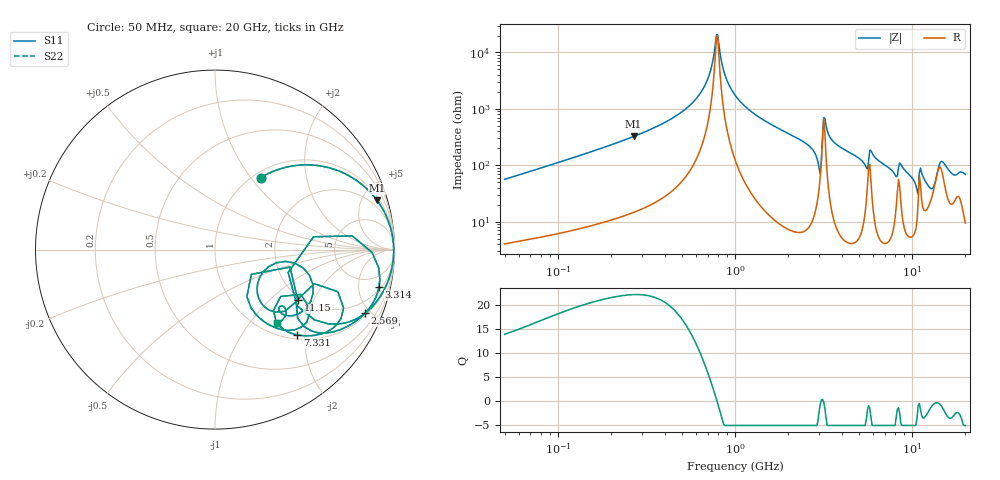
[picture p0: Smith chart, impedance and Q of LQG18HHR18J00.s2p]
!Murata Part Number: LQG18HHR18J00
!These Parameters are Measured in Series Mode Connection
!  o--[Z]--o
!Port1  Port2
!  o-------o
!Freq. Start=50[MHz] Stop=20[GHz], 401[Steps]
# Hz S RI R 50
!Freq.(Hz) S11(Real) S11(Imag) S21(Real) S21(Imag) S12(Real) S12(Imag) S22(Real) S22(Imag)
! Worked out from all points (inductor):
!   401 points, 50 MHz to 20 GHz, reference 50 ohm
!   read as one part in series: L = 176 nH near 51.52 MHz
!   highest Q = 22.2 at 267.6 MHz (marker M1), where L = 192 nH
!   self-resonance near 786.9 MHz
!   S11 on the Smith chart (normalised r, x): 50 MHz: 1.08, +1.12; 2.569 GHz: 1.15, -4.63; 3.314 GHz: 2.41, -8.24; 7.331 GHz: 1.09, -1.83; 11.15 GHz: 1.91, -1.53; 20 GHz: 1.19, -1.37
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5e7  0.2552 0.4016  0.7448 -0.4016  0.7448 -0.4016  0.2552 0.4016
1.364002e8  0.6917 0.4374  0.3083 -0.4374  0.3083 -0.4374  0.6917 0.4374
2.676374e8  0.9027 0.2747  0.0973 -0.2747  0.0973 -0.2747  0.9027 0.2747
3.721004e8  0.9546 0.1859  0.0454 -0.1859  0.0454 -0.1859  0.9546 0.1859
6.380365e8  0.9921 0.0514  0.00789 -0.0514  0.00789 -0.0514  0.9921 0.0514
7.192613e8  0.9947 0.0229  0.0053 -0.0229  0.0053 -0.0229  0.9947 0.0229
7.868965e8  0.9955 0.00159  0.0045 -0.00159  0.0045 -0.00159  0.9955 0.00159
1e9  0.9928 -0.0561  0.00721 0.0561  0.00721 0.0561  0.9928 -0.0561
2.569357e9  0.8352 -0.3553  0.1648 0.3553  0.1648 0.3553  0.8352 -0.3553
2.728004e9  0.7778 -0.3905  0.2222 0.3905  0.2222 0.3905  0.7778 -0.3905
2.98453e9  0.4577 -0.3134  0.5423 0.3134  0.5423 0.3134  0.4577 -0.3134
3.121702e9  0.7642 0.0764  0.2358 -0.0764  0.2358 -0.0764  0.7642 0.0764
3.314454e9  0.9142 -0.2071  0.0858 0.2071  0.0858 0.2071  0.9142 -0.2071
4.026975e9  0.7937 -0.3921  0.2063 0.3921  0.2063 0.3921  0.7937 -0.3921
5.769027e9  0.6845 -0.2348  0.3155 0.2348  0.3155 0.2348  0.6845 -0.2348
7.331367e9  0.4592 -0.4753  0.5408 0.4753  0.5408 0.4753  0.4592 -0.4753
7.442007e9  0.4423 -0.4714  0.5577 0.4714  0.5577 0.4714  0.4423 -0.4714
1.050288e10  0.202 -0.3261  0.798 0.3261  0.798 0.3261  0.202 -0.3261
1.115139e10  0.4618 -0.2827  0.5382 0.2827  0.5382 0.2827  0.4618 -0.2827
1.375312e10  0.392 -0.0657  0.608 0.0657  0.608 0.0657  0.392 -0.0657
1.573793e10  0.4631 -0.3588  0.5369 0.3588  0.5369 0.3588  0.4631 -0.3588
2e10  0.3435 -0.4113  0.6565 0.4113  0.6565 0.4113  0.3435 -0.4113
